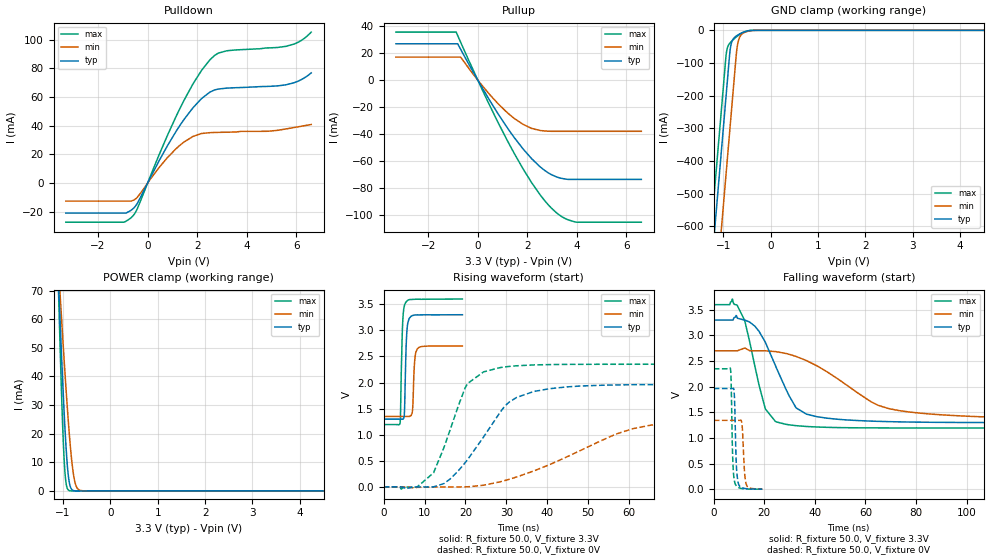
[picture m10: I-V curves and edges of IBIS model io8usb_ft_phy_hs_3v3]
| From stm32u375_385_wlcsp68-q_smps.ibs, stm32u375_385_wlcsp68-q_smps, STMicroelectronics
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[Model]   io8usb_ft_phy_hs_3v3
Model_type I/O
Polarity   Non-Inverting
Enable   Active-Low
| CAP_THRESHOLD on pad DPFT is "UDTCAPC" :
| Rising=30.0% of vddiom   Falling=70.0% of vddiom
| C_comp min and max val. don't necessarily correlate with the min and max pvt
| but are the smallest and greatest pad capacitance found.
| var   typ   min   max
C_comp   7.90877pF  7.74428pF  7.91322pF
|C_comp_pullup   5.14447pF  4.79213pF  5.27993pF
|C_comp_pulldown   2.76430pF  2.95215pF  2.63329pF
Vinl = 1.35V
Vinh = 1.8V
Vmeas = 1.65V   | Reference voltage for timing measurements
Cref  = 50.0pF   | Timing specification test load capacitance value
Rref  = 1.0MOhm   | Timing specification test load resistance value
Vref  = 1.815V   | Timing specification test load voltage
[Model Spec]
| TIME_THRESHOLD on pin ZIUSBPV11 is "CMOS" :
| Rising=50.0% of vdd   Falling=50.0% of vdd
Vinl 1.26850V 1.05950V 1.35350V
Vinh 1.77850V 1.50350V 1.88250V
| variable   typ   min   max
[Temperature Range] 25.0 130.0 -40.0
| variable   typ   min   max
[Voltage Range] 3.3V 2.7V 3.6V
| variable   typ   min   max
[POWER Clamp Reference] 3.3V 2.7V 3.6V
| variable   typ   min   max
[GND Clamp Reference] 0V 0V 0V
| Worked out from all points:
|   slope of the pulldown table from 0 to 0.495 V, typ, clamps not added: 29.9 ohm
|   slope of the pullup table from 0 to 0.495 V, typ, clamps not added: 32 ohm
|   GND clamp passes 1 mA (typ) near -0.45 V on its own axis
|   POWER clamp passes 1 mA (typ) near -0.83 V on its own axis
|   rising waveform, R_fixture 50.0, V_fixture 3.3V: 20-80 % time 431ps typ, 436ps min, 449ps max; typ from 1.3 V to 3.3 V
|   falling waveform, R_fixture 50.0, V_fixture 3.3V: 20-80 % time 11.2ns typ, 26.1ns min, 6.76ns max; typ from 3.3 V to 1.3 V
|   rising waveform, R_fixture 50.0, V_fixture 0V: 20-80 % time 10.8ns typ, 23.9ns min, 6.58ns max; typ from 0 V to 1.96 V
|   falling waveform, R_fixture 50.0, V_fixture 0V: 20-80 % time 697ps typ, 856ps min, 643ps max; typ from 1.96 V to 0.001 V
[POWER Clamp]
-3.3V     1.126A     769.5mA    1.647A
-1.1V     75.38mA    79.63mA    73.18mA
-1.09V    71.2mA     76.8mA     67.14mA
-1.08V    67.05mA    73.98mA    61.2mA
-1.06V    58.89mA    68.38mA    49.67mA
-1.01V    39.47mA    54.71mA    24.03mA
-970mV    25.49mA    44.18mA    9.257mA
-930mV    13.81mA    34.16mA    2.168mA
-870mV    3.251mA    20.56mA    140.6uA
-760mV    67.19uA    3.98mA     740.2nA
-630mV    519.2nA    149uA      2.216nA
6.6V      0A         0A         0A
[GND Clamp]
-3.3V     -4.213A    -4.451A    -4.087A
-1.25V    -727.6mA   -966.1mA   -601.9mA
-950mV    -217.6mA   -456.1mA   -91.89mA
-930mV    -183.6mA   -422.1mA   -65.18mA
-860mV    -66.05mA   -303.1mA   -39.14mA
-840mV    -46.26mA   -269.1mA   -35.85mA
-800mV    -28.83mA   -201.1mA   -30.02mA
-720mV    -16.98mA   -67.05mA   -19.74mA
-670mV    -12.46mA   -27.4mA    -14.18mA
-590mV    -6.767mA   -9.636mA   -7.036mA
-220mV    -696.1nA   -13.77uA   -55.48nA
6.6V      4.659nA    635.5nA    2.057nA
| variable   typ   min   max
[Pullup Reference] 3.3V 2.7V 3.6V
| variable   typ   min   max
[Pulldown Reference] 0V 0V 0V
[Pullup]
-3.3V     26.97mA    17.04mA    35.66mA
-870mV    26.97mA    17.04mA    35.66mA
-810mV    26.97mA    17.04mA    33.13mA
-690mV    22.87mA    17.04mA    28.11mA
460mV     -14.44mA   -10.33mA   -18.04mA
1.48V     -42.93mA   -28.64mA   -54.8mA
2.17V     -58.4mA    -35.95mA   -76.19mA
2.51V     -64.43mA   -37.5mA    -85.2mA
3.23V     -72.37mA   -38.12mA   -99.5mA
3.6V      -73.79mA   -38.12mA   -103.6mA
3.99V     -73.9mA    -38.12mA   -105.7mA
6.6V      -73.9mA    -38.12mA   -105.7mA
[Pulldown]
-3.3V     -20.86mA   -12.55mA   -27.21mA
-950mV    -20.86mA   -12.55mA   -27.21mA
-570mV    -17.52mA   -11.93mA   -22.39mA
-410mV    -13.94mA   -9.786mA   -17.62mA
800mV     26.03mA    17.78mA    33.27mA
1.3V      40.06mA    26.28mA    51.85mA
2.17V     58.78mA    34.54mA    78.34mA
2.7V      64.86mA    35.26mA    88.9mA
3.19V     66.13mA    35.45mA    92.13mA
5.58V     68.45mA    37.72mA    95.24mA
6.13V     71.47mA    39.39mA    98.65mA
6.6V      76.78mA    40.81mA    105.2mA
[Ramp]
dV/dt_r 1.17825V/10.75531ns 805.50959mV/23.63148ns 1.4097V/6.47412ns
dV/dt_f 1.2009V/11.03577ns 808.36658mV/25.87155ns 1.44328V/6.6334ns
R_load = 50.0
| Removed startup time: 0s 0s 0s  .
| Removed end time: 19.25ns.
[Rising Waveform]
R_fixture   = 50.0
V_fixture   = 3.3V
V_fixture_min = 2.7V
V_fixture_max = 3.6V
0s        1.298V     1.35V      1.195V
4ns       1.299V     1.35V      1.22V
4.65ns    1.297V     1.35V      3.142V
5.1ns     1.456V     1.35V      3.479V
5.4ns     2.433V     1.35V      3.532V
5.85ns    3.114V     1.35V      3.571V
7ns       3.28V      1.434V     3.591V
7.6ns     3.292V     2.426V     3.594V
8.25ns    3.295V     2.646V     3.595V
19.25ns   3.298V     2.698V     3.598V
| Removed startup time: 0s 0s 0s  .
| Removed end time: 199.25ns.
[Falling Waveform]
R_fixture   = 50.0
V_fixture   = 3.3V
V_fixture_min = 2.7V
V_fixture_max = 3.6V
0s        3.3V       2.7V       3.6V
7.35ns    3.3V       2.7V       3.709V
9.3ns     3.336V     2.7V       3.584V
12.3ns    3.299V     2.754V     3.278V
20.4ns    2.867V     2.7V       1.566V
28.45ns   1.962V     2.649V     1.266V
32.55ns   1.587V     2.59V      1.239V
36.6ns    1.465V     2.511V     1.224V
73.2ns    1.314V     1.534V     1.195V
199.3ns   1.298V     1.353V     1.195V
| Removed startup time: 0s 0s 0s  .
| Removed end time: 199.25ns.
[Rising Waveform]
R_fixture   = 50.0
V_fixture   = 0V
V_fixture_min = 0V
V_fixture_max = 0V
0s        35.01nV    299.5nV    81.69nV
8.15ns    -588.7uV   -7.979mV   -3.646mV
12.2ns    659.8uV    -702.7uV   270.6mV
20.35ns   506.5mV    2.021mV    1.958V
28.8ns    1.464V     104.8mV    2.289V
32.55ns   1.716V     191.3mV    2.32V
40.65ns   1.882V     430mV      2.343V
56.95ns   1.953V     1.016V     2.349V
73.2ns    1.962V     1.252V     2.349V
199.3ns   1.964V     1.343V     2.349V
| Removed startup time: 0s 0s 0s  .
| Removed end time: 19.2ns.
[Falling Waveform]
R_fixture   = 50.0
V_fixture   = 0V
V_fixture_min = 0V
V_fixture_max = 0V
0s        1.964V     1.343V     2.349V
6.6ns     1.964V     1.343V     2.348V
7.55ns    1.964V     1.343V     532.9mV
8.1ns     1.866V     1.343V     180.8mV
8.45ns    1.331V     1.343V     108.7mV
9ns       412.6mV    1.343V     60.78mV
9.8ns     97.57mV    1.343V     32.08mV
11.2ns    27.57mV    1.25V      11.93mV
12.95ns   9.325mV    79.51mV    4.397mV
19.2ns    1.343mV    2.285mV    371.1uV
